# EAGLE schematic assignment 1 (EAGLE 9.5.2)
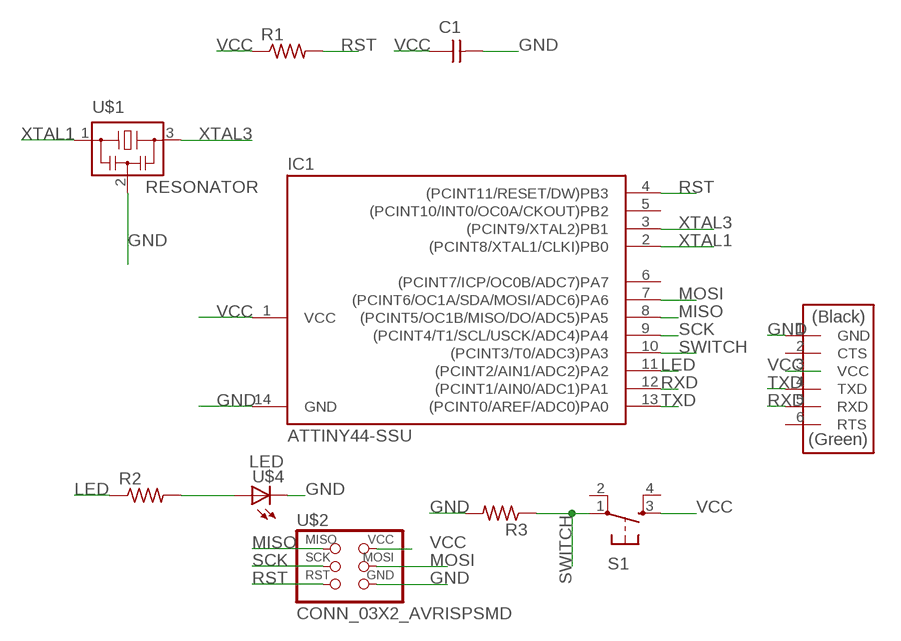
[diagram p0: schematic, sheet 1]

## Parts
C1  CAP-UNPOLARIZEDFAB  [C1206FAB]
IC1  ATTINY44-SSU  [SOIC14]
R1  R1206FAB  [R1206FAB]
R2  RES-US1206FAB  [R1206FAB]
R3  R1206FAB  [R1206FAB]
S1  6MM_SWITCH6MM_SWITCH  [6MM_SWITCH]
U$1  RESONATOR  [EFOBM]
U$2  CONN_03X2_AVRISPSMD  [2X03SMD]
U$3  CONN_06_FTDI-SMD-HEADER  [1X06SMD]
U$4  LED  [LED1206]

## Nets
GND: C1.2 IC1.14(GND) R3.2 U$1.2 U$2.6(GND) U$3.1(GND) U$4.2(C)
LED: IC1.11((PCINT2/AIN1/ADC2)PA2) R2.1
MISO: IC1.8((PCINT5/OC1B/MISO/DO/ADC5)PA5) U$2.1(MISO)
MOSI: IC1.7((PCINT6/OC1A/SDA/MOSI/ADC6)PA6) U$2.4(MOSI)
N$11: R2.2 U$4.1(A)
RST: IC1.4((PCINT11/RESET/DW)PB3) R1.2 U$2.5(RST)
RXD: IC1.12((PCINT1/AIN0/ADC1)PA1) U$3.5(RXD)
SCK: IC1.9((PCINT4/T1/SCL/USCK/ADC4)PA4) U$2.3(SCK)
SWITCH: IC1.10((PCINT3/T0/ADC3)PA3) R3.1 S1.1(P)
TXD: IC1.13((PCINT0/AREF/ADC0)PA0) U$3.4(TXD)
VCC: C1.1 IC1.1(VCC) R1.1 S1.3(S) U$2.2(VCC) U$3.3(VCC)
XTAL1: IC1.2((PCINT8/XTAL1/CLKI)PB0) U$1.1
XTAL3: IC1.3((PCINT9/XTAL2)PB1) U$1.3
Unconnected: IC1.5((PCINT10/INT0/OC0A/CKOUT)PB2) IC1.6((PCINT7/ICP/OC0B/ADC7)PA7) S1.2(P1) S1.4(S1) U$3.2(CTS) U$3.6(RTS)

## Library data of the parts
C1 = fab:CAP-UNPOLARIZED
IC1 = fab:ATTINY44
R1 R3 = fab:R: Resistor (US Symbol)
R2 = fab:RES-US: Resistor (US Symbol)
S1 = fab:6MM_SWITCH: OMRON SWITCH
U$1 = fab:RESONATOR
U$2 = fab:CONN_03X2_AVRISP
U$3 = fab:CONN_06_FTDI-SMD-HEADER
U$4 = fab:LED: LED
